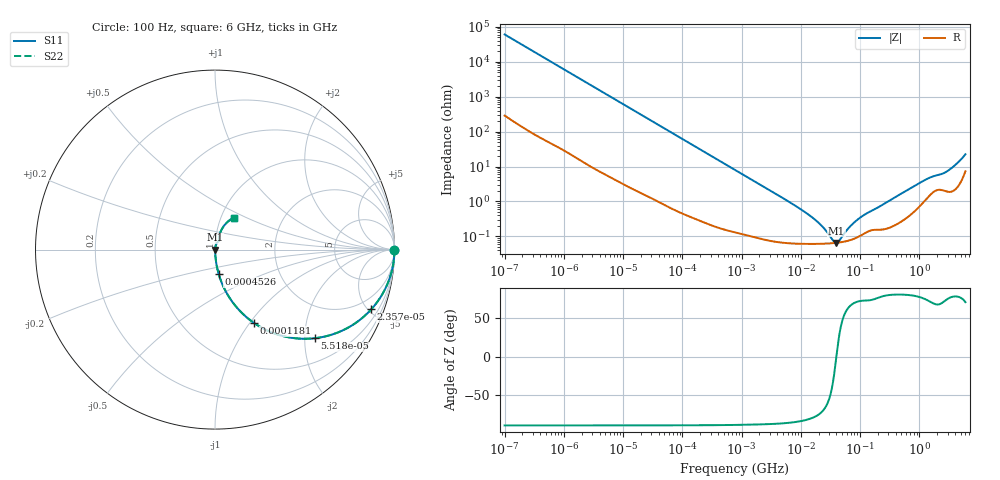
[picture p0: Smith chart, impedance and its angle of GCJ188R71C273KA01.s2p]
!Murata Part Number: GCJ188R71C273KA01
!These Parameters are Measured in Series Mode Connection
!Data Generated on Mar 13, 2026
!  o--ll--o
!Port1  Port2
!  o------o
!Operation Temp=25[degC], DC Bias Voltage=0[V]
!Freq. Start=100[Hz] Stop=6[GHz] 401[Steps]
# Hz S RI R 50
!Freq.(Hz) S11(Real) S11(Imag) S21(Real) S21(Imag) S12(Real) S12(Imag) S22(Real) S22(Imag)
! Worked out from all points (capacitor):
!   401 points, 100 Hz to 6 GHz, reference 50 ohm
!   read as one part in series: C = 26.3 nF near 109 Hz
!   lowest |Z| = 65.2 mohm at 39.84 MHz (marker M1)
!   series resonance near 39.85 MHz, so ESL is about 610 pH
!   S11 on the Smith chart (normalised r, x): 100 Hz: open; 23.57 kHz: 1.03, -5.22; 55.18 kHz: 1.01, -2.24; 118.1 kHz: 1.01, -1.05; 452.6 kHz: 1.00, -0.27; 6 GHz: 1.15, +0.42
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100  1 -0.00165  1.06e-05 0.00165  1.06e-05 0.00165  1 -0.00165
2008  0.9988 -0.0329  0.00123 0.0329  0.00123 0.0329  0.9988 -0.0329
8047  0.9824 -0.1289  0.0176 0.1289  0.0176 0.1289  0.9824 -0.1289
23569  0.8705 -0.3329  0.1295 0.3329  0.1295 0.3329  0.8705 -0.3329
40335  0.6989 -0.4556  0.3011 0.4556  0.3011 0.4556  0.6989 -0.4556
55182  0.5552 -0.4937  0.4448 0.4937  0.4448 0.4937  0.5552 -0.4937
118133  0.217 -0.4084  0.783 0.4084  0.783 0.4084  0.217 -0.4084
211427  0.0813 -0.2688  0.9187 0.2688  0.9187 0.2688  0.0813 -0.2688
452617  0.0201 -0.1345  0.9799 0.1345  0.9799 0.1345  0.0201 -0.1345
774597  0.00772 -0.0798  0.9923 0.0798  0.9923 0.0798  0.00772 -0.0798
6353432  0.000727 -0.00968  0.9993 0.00968  0.9993 0.00968  0.000727 -0.00968
1.555665e7  0.000619 -0.00344  0.9994 0.00344  0.9994 0.00344  0.000619 -0.00344
2.327686e7  0.000617 -0.00179  0.9994 0.00179  0.9994 0.00179  0.000617 -0.00179
3.482834e7  0.000638 -0.000428  0.9994 0.000428  0.9994 0.000428  0.000638 -0.000428
3.983537e7  0.000652 -1.4e-06  0.9993 1.4e-06  0.9993 1.4e-06  0.000652 -1.4e-06
4.556224e7  0.000671 0.000425  0.9993 -0.000425  0.9993 -0.000425  0.000671 0.000425
6.817316e7  0.000782 0.00177  0.9992 -0.00177  0.9992 -0.00177  0.000782 0.00177
9.326766e7  0.000975 0.00297  0.999 -0.00297  0.999 -0.00297  0.000975 0.00297
3.124326e8  0.00186 0.0104  0.9981 -0.0104  0.9981 -0.0104  0.00186 0.0104
1.309207e9  0.0131 0.0403  0.9869 -0.0403  0.9869 -0.0403  0.0131 0.0403
2.802721e9  0.0233 0.0637  0.9767 -0.0637  0.9767 -0.0637  0.0233 0.0637
6e9  0.1031 0.1775  0.8969 -0.1775  0.8969 -0.1775  0.1031 0.1775
